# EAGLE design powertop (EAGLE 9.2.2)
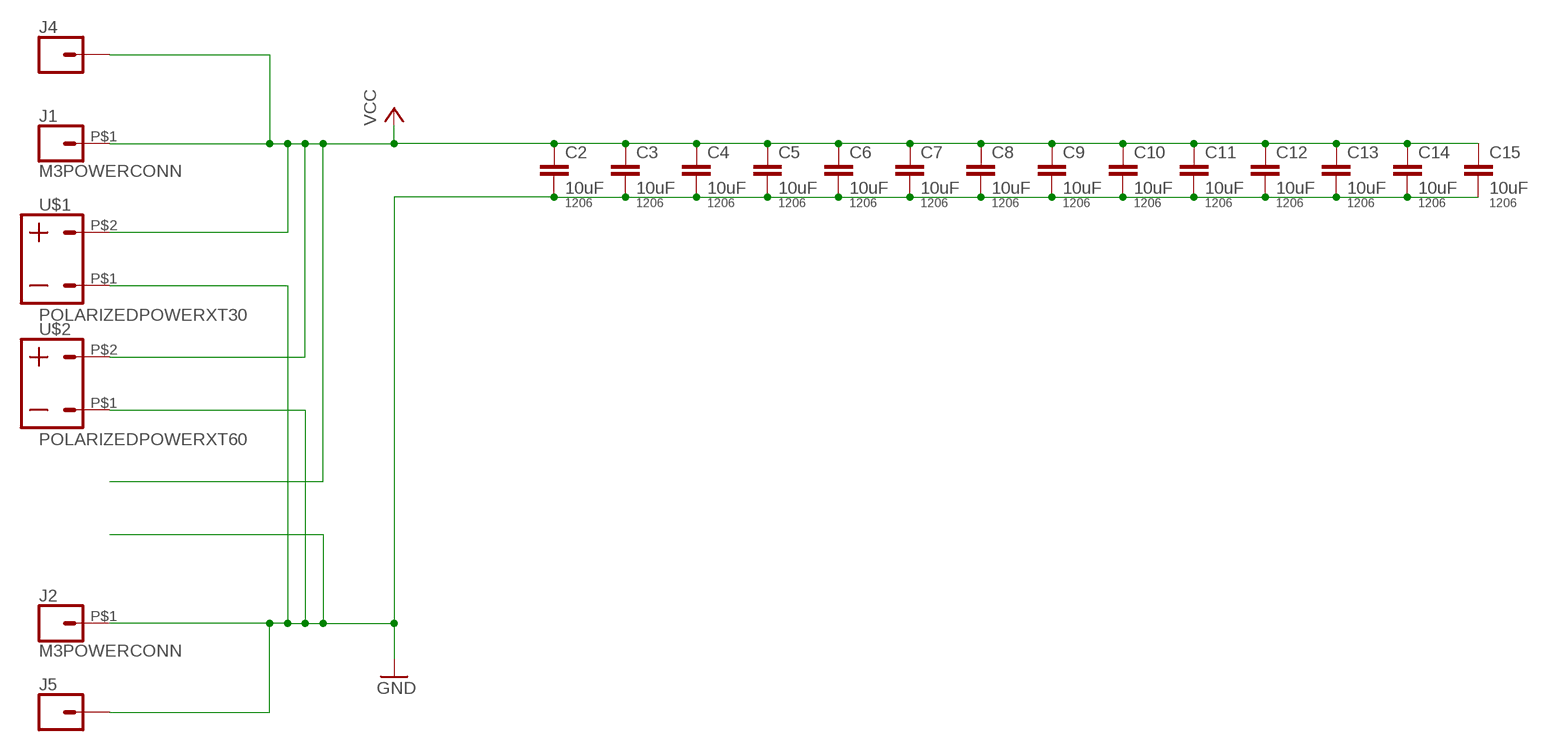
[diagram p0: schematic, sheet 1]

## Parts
C2  10uF  CAP1206  [1206]
C3  10uF  CAP1206  [1206]
C4  10uF  CAP1206  [1206]
C5  10uF  CAP1206  [1206]
C6  10uF  CAP1206  [1206]
C7  10uF  CAP1206  [1206]
C8  10uF  CAP1206  [1206]
C9  10uF  CAP1206  [1206]
C10  10uF  CAP1206  [1206]
C11  10uF  CAP1206  [1206]
C12  10uF  CAP1206  [1206]
C13  10uF  CAP1206  [1206]
C14  10uF  CAP1206  [1206]
C15  10uF  CAP1206  [1206]
J1  M3POWERCONN  [M3POWERCONN]
J2  M3POWERCONN  [M3POWERCONN]
J4  CONN_01OFFSET  [1X01_OFFSET]
J5  CONN_01OFFSET  [1X01_OFFSET]
U$1  POLARIZEDPOWERXT30  [XT30]
U$2  POLARIZEDPOWERXT60  [XT60]

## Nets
GND: C2.2 C3.2 C4.2 C5.2 C6.2 C7.2 C8.2 C9.2 C10.2 C11.2 C12.2 C13.2 C14.2 C15.2 J2.P$1 J5.1 U$1.P$1 U$2.P$1
VCC: C2.1 C3.1 C4.1 C5.1 C6.1 C7.1 C8.1 C9.1 C10.1 C11.1 C12.1 C13.1 C14.1 C15.1 J1.P$1 J4.1 U$1.P$2 U$2.P$2

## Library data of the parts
C2-C15 = passives:CAP: Capacitor; PACKAGE: 1206
J1 J2 = connector:M3POWERCONN
J4 J5 = SparkFun-Connectors:CONN_01: Single connection point. Often used as Generic Header-pin footprint for 0.1 inch spaced/style header connections
U$1 U$2 = connector:POLARIZEDPOWER

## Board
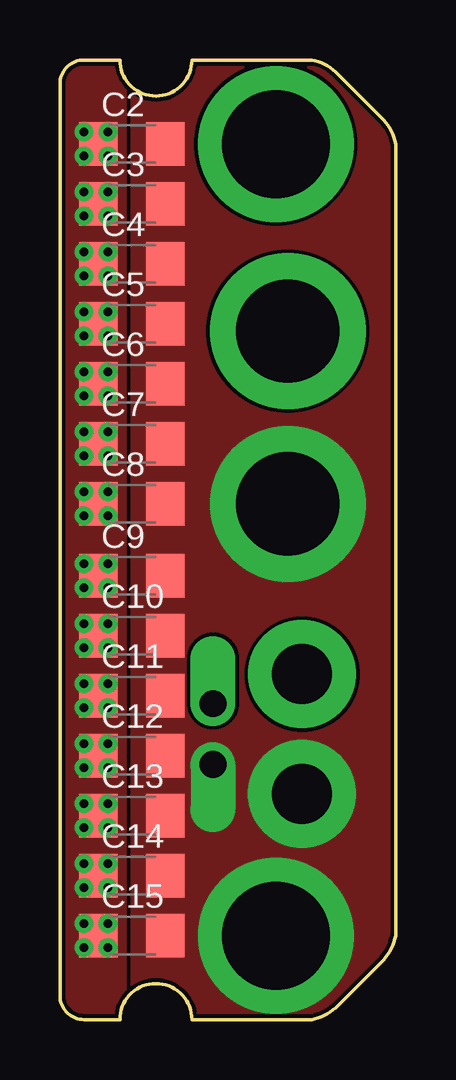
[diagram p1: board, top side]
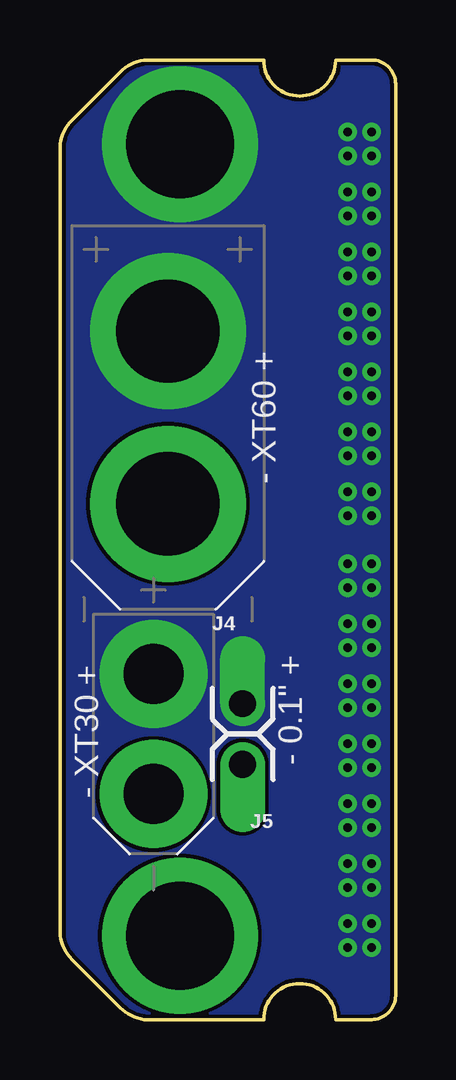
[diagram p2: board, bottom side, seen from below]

Size 14 x 40 mm. Coordinates in mm from the lower left corner, seen from the top.
Outline: 13.5,37.5 arc-37 14,36.5 14,3.5 arc-37 13.5,2.5 11.5,0.5 arc-37 10.5,0 5.5,0 arc90 4,1.5 arc90 2.5,0 1,0 arc-90 0,1 0,39 arc-90 1,40 2.5,40 arc90 4,38.5 arc90 5.5,40 10.5,40 arc-37 11.5,39.5 13.5,37.5
Copper layers (1*16): Top 0.035mm / dielectric 1.5mm / Bottom 0.035mm
Design rules "default *": minimum track width 6mil, minimum drill 0.35mm, track to track 6mil, track to pad 6mil, pad to pad 6mil, via to via 6mil, smd to smd 6mil, copper to edge 6mil, drill to drill 6mil, minimum pad ring 10mil, minimum via ring 8mil, stop-mask expansion 4mil, vias tented up to drill 30mil, thermal gap 10mil

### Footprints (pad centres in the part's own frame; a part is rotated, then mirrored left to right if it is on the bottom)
1206 = smd 1.6 x 1.8: 1 -1.4,0; 2 1.4,0
M3POWERCONN = drill 4.5 pad 6.5: P$1 0,0
1X01_OFFSET = drill 1.118 pad 1.88 offset: 1 0,0
XT30 = drill 2.5 pad 4.5: P$1 2.5,0; P$2 -2.5,0
XT60 = drill 4.3 pad 6.5: P$1 3.6,0; P$2 -3.6,0

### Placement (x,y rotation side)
C2  3,36.5 0 top
C3  3,34 0 top
C4  3,31.5 0 top
C5  3,29 0 top
C6  3,26.5 0 top
C7  3,24 0 top
C8  3,21.5 0 top
C9  3,18.5 0 top
C10  3,16 0 top
C11  3,13.5 0 top
C12  3,11 0 top
C13  3,8.5 0 top
C14  3,6 0 top
C15  3,3.5 0 top
J1  9,36.5 0 top
J2  9,3.5 0 top
J4  6.38,13.17 0 bottom
J5  6.38,10.63 180 bottom
U$1  10.1,11.9 270 bottom
U$2  9.5,25.1 270 bottom

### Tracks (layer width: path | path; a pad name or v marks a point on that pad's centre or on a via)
GND
  pour Top (no thermals): 3,41 3,-1 15,-1 15,41
VCC  (via drill 0.35)
  other vias: 1,37 1,36 2,37 2,36 1,34.5 1,33.5 2,34.5 2,33.5 1,9 1,8 2,9 2,8 1,6.5 1,5.5 2,6.5 2,5.5 1,4 1,3 2,4 2,3 1,16.5 1,15.5 2,16.5 2,15.5 1,14 1,13 2,14 2,13 1,11.5 1,10.5 2,11.5 2,10.5 1,24.5 1,23.5 2,24.5 2,23.5 1,22 1,21 2,22 2,21 1,19 1,18 2,19 2,18 1,32 1,31 2,32 2,31 1,29.5 1,28.5 2,29.5 2,28.5 1,27 1,26 2,27 2,26
  pour Top (rank 2, no thermals): 3,41 -0.5,41 -0.5,-1 3,-1
  pour Bottom (rank 2, no thermals): -1,41.5 15.5,41.5 15.5,-1.5 -1,-1.5

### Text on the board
bPlace: - XT60 + | - 0.1" + | - XT30 +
